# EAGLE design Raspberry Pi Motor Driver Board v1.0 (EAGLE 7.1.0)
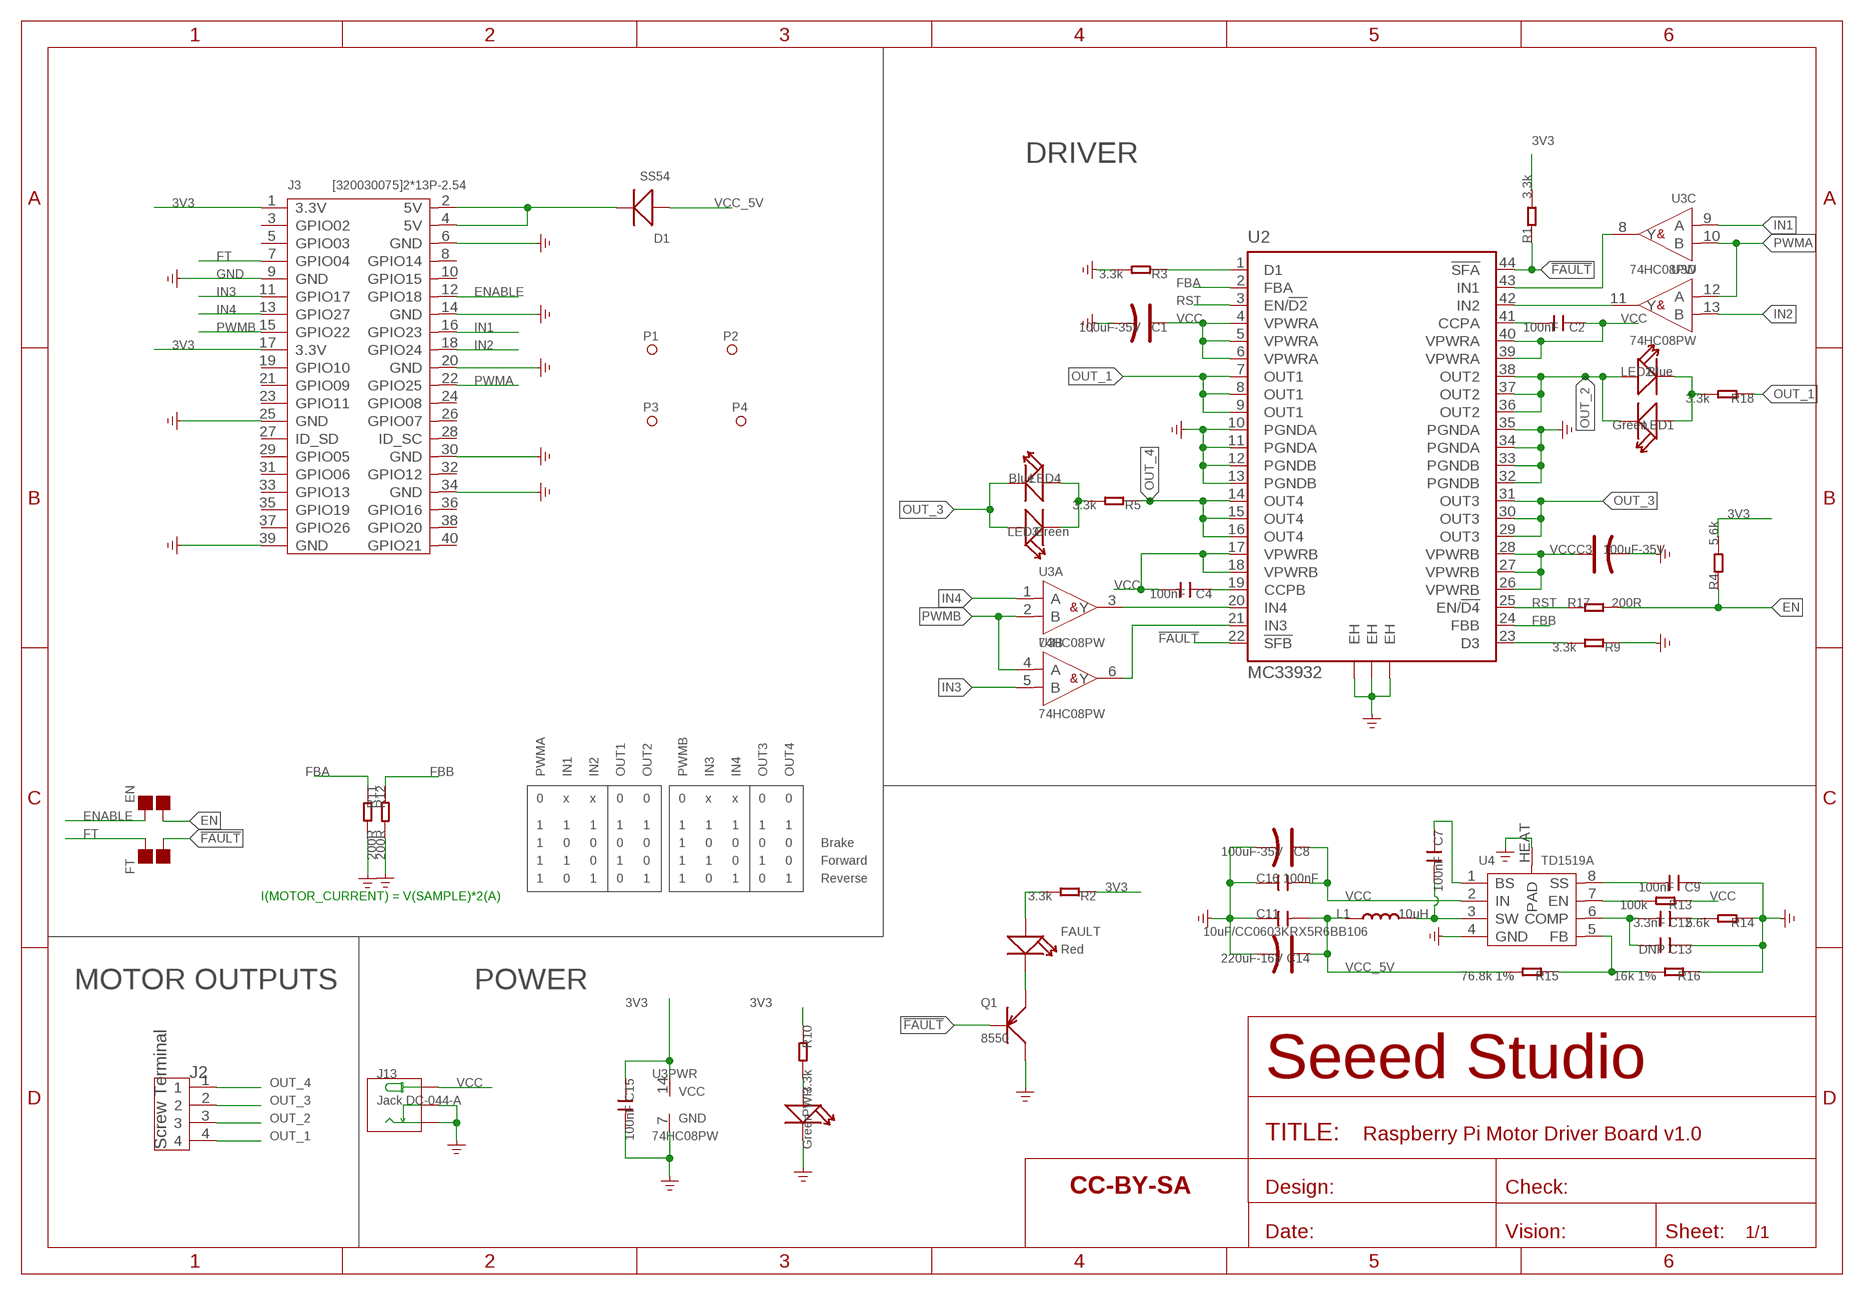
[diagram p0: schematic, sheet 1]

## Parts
C1  100uF-35V  CAP-ELECTRO-E  [ELECTRO-SMD-E-7.8MM]
C2  100nF  C-0603  [C0603]
C3  100uF-35V  CAP-ELECTRO-E  [ELECTRO-SMD-E-7.8MM]
C4  100nF  C-0603  [C0603]
C7  100nF  C-0603  [C0603]
C8  100uF-35V  CAP-ELECTRO-E  [ELECTRO-SMD-E-7.8MM]
C9  100nF  C-0603  [C0603]
C11  10uF/CC0603KRX5R6BB106  C-0603  [C0603]
C12  3.3nF  C-0603  [C0603]
C13  DNP  C-0603  [C0603]
C14  220uF-16V  CAP-ELECTRO-D  [ELECTRO-SMD-D-5.6MM]
C15  100nF  C-0603  [C0603]
C16  100nF  C-0603  [C0603]
D1  SS54  DIODESMB  [DO_214AA]
EN  PAD-JUMPER-2P  [2P-SMD-1.78X1.27]
FAULT  Red  LED'0603'  [LED-0603]
FT  PAD-JUMPER-2P  [2P-SMD-1.78X1.27]
J2  Screw Terminal  SCREW-TERMINAL-4P'3.5'  [4P-3.5]
J3  [320030075]2*13P-2.54  HEADER-2X20P  [2X20P-2.54-65/35MIL]
J13  Jack DC-044-A  JACK-DC-044  [DC-044]
L1  10uH  L'0630'  [L0630]
LED1  Green  LED'0603'  [LED-0603]
LED2  Blue  LED'0603'  [LED-0603]
LED3  Green  LED'0603'  [LED-0603]
LED4  Blue  LED'0603'  [LED-0603]
P1  PAD-MARK'ANNULAR'  [ROUND-MARK-1.0]
P2  PAD-MARK'ANNULAR'  [ROUND-MARK-1.0]
P3  PAD-MARK'ANNULAR'  [ROUND-MARK-1.0]
P4  PAD-MARK'ANNULAR'  [ROUND-MARK-1.0]
PWR  Green  LED'0603'  [LED-0603]
Q1  8550  TRANSISTOR-PNP-SOT23  [SOT-23]
R1  3.3k  R-0603  [R0603]
R2  3.3k  R-0603  [R0603]
R3  3.3k  R-0603  [R0603]
R4  5.6k  R-0603  [R0603]
R5  3.3k  R-0603  [R0603]
R9  3.3k  R-0603  [R0603]
R10  3.3k  R-0603  [R0603]
R11  200R  R-0603  [R0603]
R12  200R  R-0603  [R0603]
R13  100k  R-0603  [R0603]
R14  5.6k  R-0603  [R0603]
R15  76.8k 1%  R-0603  [R0603]
R16  16k 1%  R-0603  [R0603]
R17  200R  R-0603  [R0603]
R18  3.3k  R-0603  [R0603]
U2  MC33932  [HSOP44]
U3  74HC08PW  [TSSOP14]
U4  TD1519A  TD1484A  [SOP8-W/HEAT]
U$12  SEEEDSTUDIO-OPEN-SCH-FRAME  [SEEEDSTUDIO-PCB-FRAME]

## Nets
3V3: C15.1 J3.1(3.3V) J3.17(3.3V) R1.2 R2.1 R4.2 R10.1 U3.14(PWR:VCC)
!FAULT: FT.1 Q1.1(B) R1.1 U2.22(!SFB) U2.44(!SFA)
EN: EN.1 R4.1 R17.2
ENABLE: EN.2 J3.12(GPIO18)
FBA: R11.1 U2.2(FBA)
FBB: R12.1 U2.24(FBB)
FT: FT.2 J3.7(GPIO04)
GND: C1.- C3.- C8.- C9.1 C11.1 C13.1 C14.- C15.2 C16.1 J3.6(GND) J3.9(GND) J3.14(GND) J3.20(GND) J3.25(GND) J3.30(GND) J3.34(GND) J3.39(GND) J13.- J13.CDN PWR.- Q1.3(C) R3.2 R9.1 R11.2 R12.2 R14.1 R16.1 U2.10(PGNDA) U2.11(PGNDA) U2.12(PGNDB) U2.13(PGNDB) U2.32(PGNDB) U2.33(PGNDB) U2.34(PGNDA) U2.35(PGNDA) U2.EH@1(EH) U2.EH@2(EH) U2.EH@3(EH) U3.7(PWR:GND) U4.4(GND) U4.HEAT(PAD) ; supply symbol labelled GND_POWER
IN1: J3.16(GPIO23) U3.9(C:A)
IN2: J3.18(GPIO24) U3.13(D:B)
IN3: J3.11(GPIO17) U3.5(B:B)
IN4: J3.13(GPIO27) U3.1(A:A)
N$1: FAULT.- Q1.2(E)
N$2: FAULT.+ R2.2
N$3: D1.2(-) J3.2(5V) J3.4(5V)
N$4: R3.1 U2.1(D1)
N$6: U2.21(IN3) U3.6(B:Y)
N$8: LED3.- LED4.+ R5.2
N$11: C7.2 L1.2 U4.3(SW)
N$12: U2.42(IN2) U3.11(D:Y)
N$14: LED1.+ LED2.- R18.2
N$15: R15.1 R16.2 U4.5(FB)
N$16: R9.2 U2.23(D3)
N$17: C9.2 U4.8(SS)
N$18: R13.2 U4.7(EN)
N$19: C7.1 U4.1(BS)
N$20: C12.2 C13.2 U4.6(COMP)
N$23: U2.43(IN1) U3.8(C:Y)
N$25: C12.1 R14.2
N$26: U2.20(IN4) U3.3(A:Y)
N$28: C2.2 U2.41(CCPA)
N$30: C4.1 U2.19(CCPB)
N$54: PWR.+ R10.2
OUT_1: J2.4 R18.1 U2.7(OUT1) U2.8(OUT1) U2.9(OUT1)
OUT_2: J2.3 LED1.- LED2.+ U2.36(OUT2) U2.37(OUT2) U2.38(OUT2)
OUT_3: J2.2 LED3.+ LED4.- U2.29(OUT3) U2.30(OUT3) U2.31(OUT3)
OUT_4: J2.1 R5.1 U2.14(OUT4) U2.15(OUT4) U2.16(OUT4)
PWMA: J3.22(GPIO25) U3.10(C:B) U3.12(D:A)
PWMB: J3.15(GPIO22) U3.2(A:B) U3.4(B:A)
RST: R17.1 U2.3(EN/!D2) U2.25(EN/!D4)
VCC: C1.+ C2.1 C3.+ C4.2 C8.+ C16.2 J13.+ R13.1 U2.4(VPWRA) U2.5(VPWRA) U2.6(VPWRA) U2.17(VPWRB) U2.18(VPWRB) U2.26(VPWRB) U2.27(VPWRB) U2.28(VPWRB) U2.39(VPWRA) U2.40(VPWRA) U4.2(IN)
VCC_5V: C11.2 C14.+ D1.1(+) L1.1 R15.2
Unconnected: J3.3(GPIO02) J3.5(GPIO03) J3.8(GPIO14) J3.10(GPIO15) J3.19(GPIO10) J3.21(GPIO09) J3.23(GPIO11) J3.24(GPIO08) J3.26(GPIO07) J3.27(ID_SD) J3.28(ID_SC) J3.29(GPIO05) J3.31(GPIO06) J3.32(GPIO12) J3.33(GPIO13) J3.35(GPIO19) J3.36(GPIO16) J3.37(GPIO26) J3.38(GPIO20) J3.40(GPIO21)

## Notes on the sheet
- DRIVER
- PWMA | IN1 | IN2 | OUT1 | OUT2 | PWMB | IN3 | IN4 | OUT3 | OUT4
- 0 | x | x | 0 | 0 | 0 | x | x | 0 | 0
- 1 | 1 | 1 | 1 | 1 | 1 | 1 | 1 | 1 | 1
- 1 | 0 | 0 | 0 | 0 | 1 | 0 | 0 | 0 | 0 | Brake
- 1 | 1 | 0 | 1 | 0 | 1 | 1 | 0 | 1 | 0 | Forward
- 1 | 0 | 1 | 0 | 1 | 1 | 0 | 1 | 0 | 1 | Reverse
- I(MOTOR_CURRENT) = V(SAMPLE)*2(A)
- MOTOR OUTPUTS | POWER

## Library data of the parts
C1 C3 C8 C14 = Discrete:CAP*: Electrolytic Capacitors,Tantalum Capacitors and Super Capacitors
C2 C4 C7 C9 C11-C13 C15 C16 = Discrete:C*: Ceramic Capacitors
D1 = Discrete-new:DIODE*
EN FT = Discrete:PAD-JUMPER-2P; PARTNO: DNP
FAULT LED1-LED4 PWR = Discrete:LED*
J2 = Connector :SCREW-TERMINAL-4P
J3 = Connector-new:HEADER-2X20P
J13 = Connector :JACK-DC-044
L1 = Discrete:L*
P1-P4 = Discrete-new:PAD-MARK; PARTNO: DNP
Q1 = Discrete-new:TRANSISTOR-PNP*: PNP audion
R1-R5 R9-R18 = Discrete:R*
U2 = template:MC33932: 5.0 A Throttle Control H-Bridge Auto generated by make-symbol-device-package-bsdl.ulp Rev. 33 Source: http://www.freescale.com/files/analog/doc/data_sheet/MC33932.pdf?fpsp=1; MPN: MC33932VW; OC_FARNELL: 1701639; OC_NEWARK: 67P3304
U3 = template :74*08: Quad 2-input AND gate
U4 = template:TD1484A: The TD1484 is a monolithic synchronous buck regulator. The device integrates two 90mΩ MOSFETs, and provides 3A of continuous load current over a wide input voltage of 4.75V to 23V. Current mode control provides fast transient response and cycle-by-cycle current limit. An adjustable soft-start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
U$12 = moudle-new:SEEEDSTUDIO-OPEN-SCH-FRAME

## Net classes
0 default: width 0.076 mm, drill 0.102 mm, clearance 0.076 mm
1 vcc: width 5.08 mm, clearance 0.254 mm

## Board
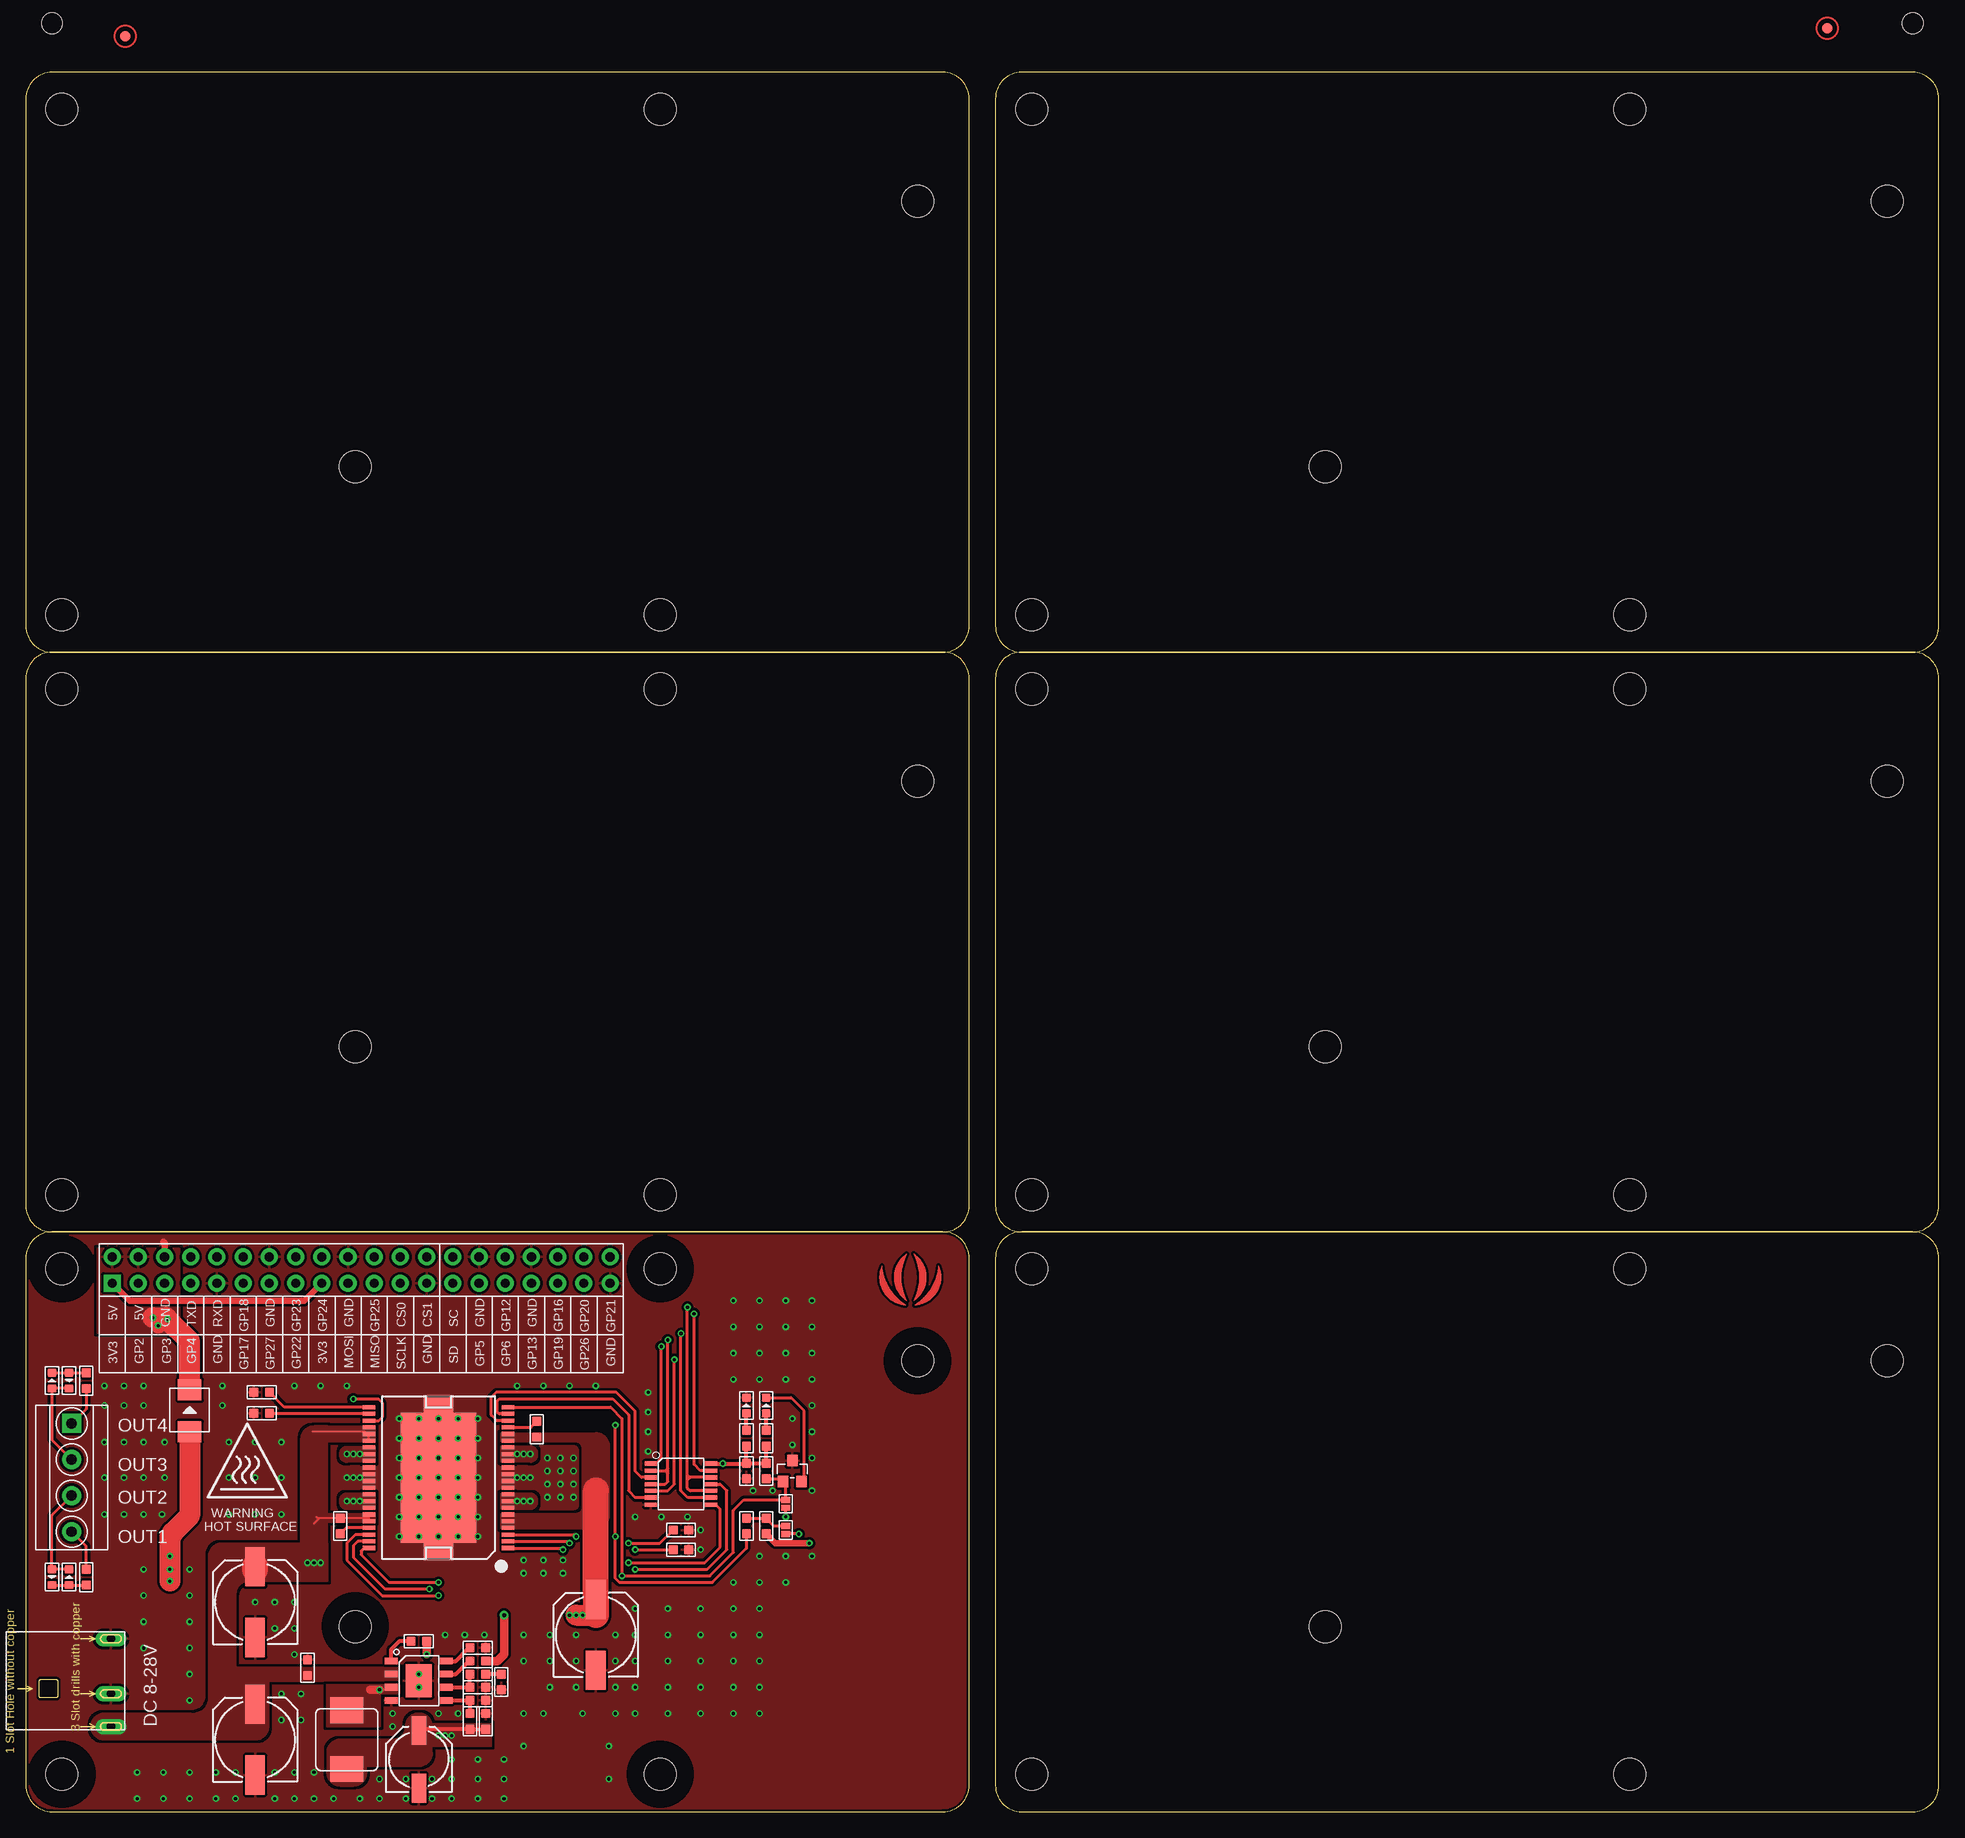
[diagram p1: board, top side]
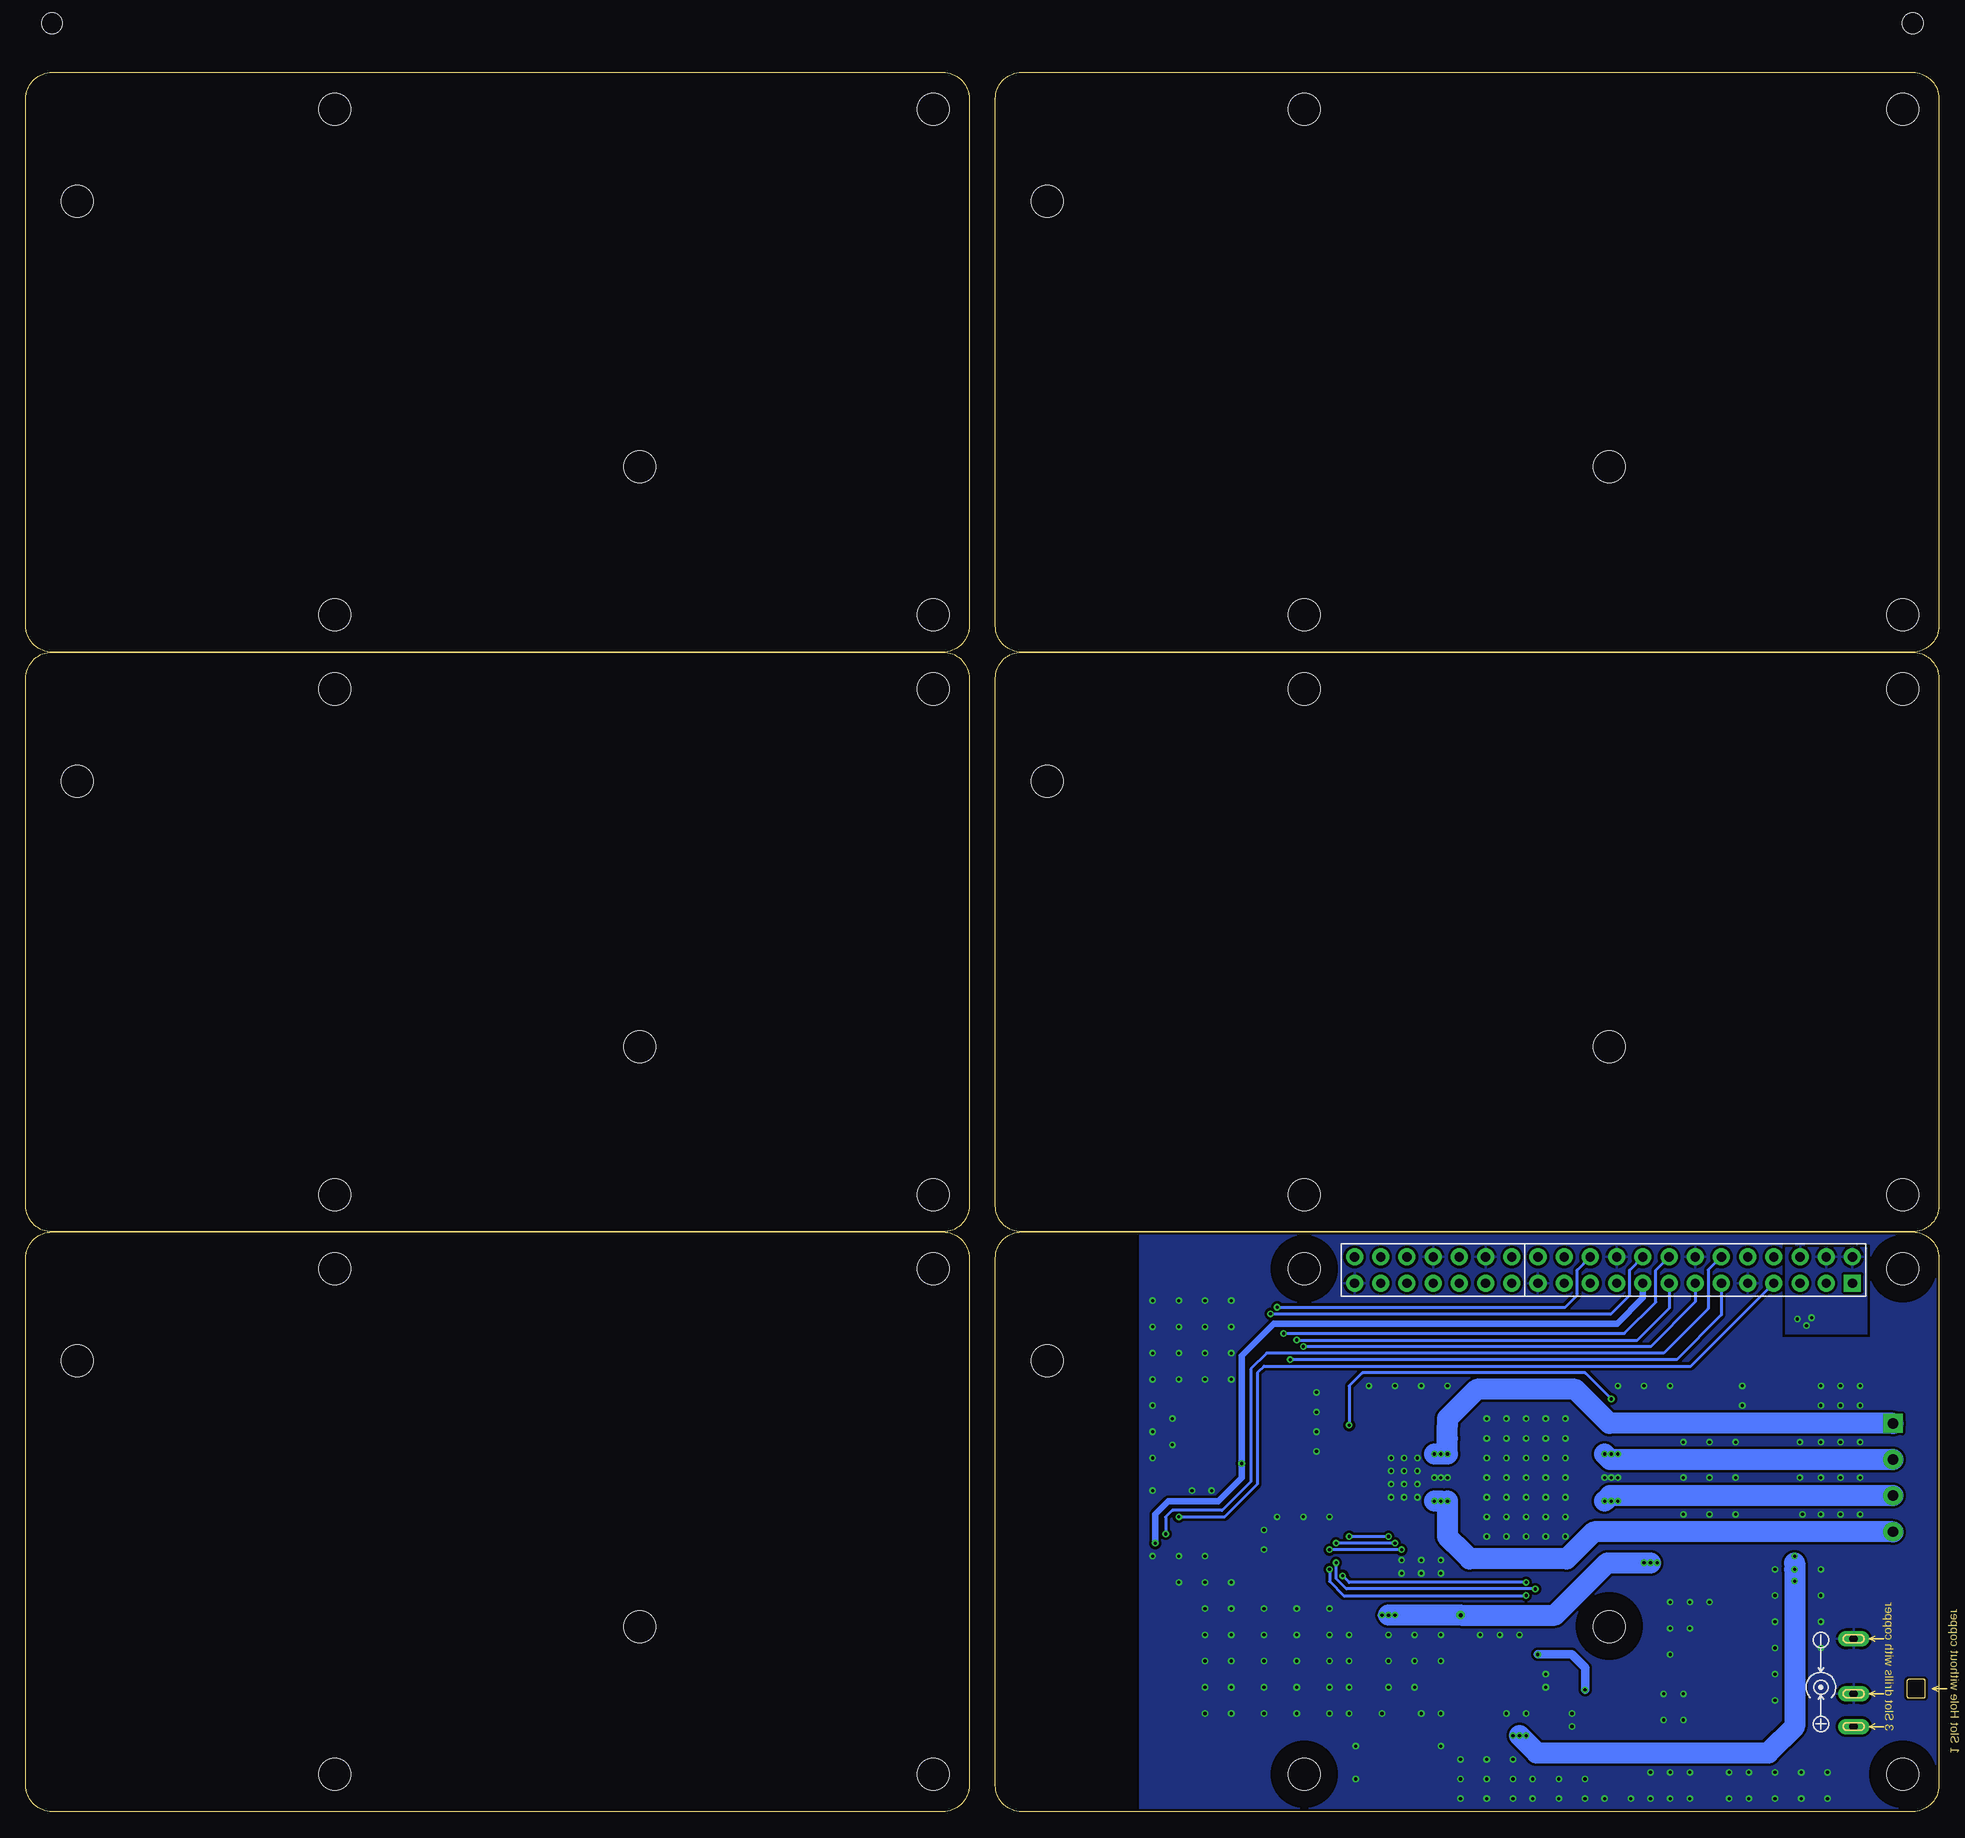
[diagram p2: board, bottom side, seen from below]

Size 185.42 x 168.59 mm. Coordinates in mm from the lower left corner, seen from the top.
Copper layers (1*16): Top 0.035mm / dielectric 1.5mm / Bottom 0.035mm
Design rules "SeeedStudio_2layer_DRU_no_angle_20140221 *": minimum track width 6mil, minimum drill 12mil, track to track 6mil, track to pad 6mil, pad to pad 6mil, via to via 6mil, smd to smd 0mil, copper to edge 10mil, drill to drill 10mil, minimum pad ring 10mil, minimum via ring 6mil, stop-mask expansion 2mil, vias tented up to drill 25mil, thermal gap 10mil
Holes 2.03 mm at 2.54,-4.45 182.88,-4.45 182.88,173.35 2.54,173.35

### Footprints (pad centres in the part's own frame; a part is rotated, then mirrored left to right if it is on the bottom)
ELECTRO-SMD-E-7.8MM = smd 3.81 x 1.905: + 3.429,0; - -3.429,0
C0603 = smd 0.889 x 0.889: 1 -0.762,0; 2 0.762,0
ELECTRO-SMD-D-5.6MM = smd 2.794 x 1.397: + 2.794,0; - -2.794,0
DO_214AA = smd 2.032 x 2.286: 1 -2.032,0; 2 2.032,0
2P-SMD-1.78X1.27 = smd 0.889 x 0.61: 1 0,0.381; 2 0,-0.381
LED-0603 = smd 0.762 x 0.889: + -0.762,0; - 0.762,0
4P-3.5 = drill 1 pad 1.85 square: 1 -5.25,0 | drill 1 pad 1.85: 2 -1.75,0; 3 1.75,0; 4 5.25,0
2X20P-2.54-65/35MIL = drill 0.889 pad 1.651 square: 1 1.27,24.13 | drill 0.889 pad 1.651: 2 -1.27,24.13; 3 1.27,21.59; 4 -1.27,21.59; 5 1.27,19.05; 6 -1.27,19.05; 7 1.27,16.51; 8 -1.27,16.51; 9 1.27,13.97; 10 -1.27,13.97; 11 1.27,11.43; 12 -1.27,11.43; 13 1.27,8.89; 14 -1.27,8.89; 15 1.27,6.35; 16 -1.27,6.35; 17 1.27,3.81; 18 -1.27,3.81; 19 1.27,1.27; 20 -1.27,1.27; 21 1.27,-1.27; 22 -1.27,-1.27; 23 1.27,-3.81; 24 -1.27,-3.81; 25 1.27,-6.35; 26 -1.27,-6.35; 27 1.27,-8.89; 28 -1.27,-8.89; 29 1.27,-11.43; 30 -1.27,-11.43; 31 1.27,-13.97; 32 -1.27,-13.97; 33 1.27,-16.51; 34 -1.27,-16.51; 35 1.27,-19.05; 36 -1.27,-19.05; 37 1.27,-21.59; 38 -1.27,-21.59; 39 1.27,-24.13; 40 -1.27,-24.13
DC-044 = drill 0.813 pad 1.524 long: + 3.175,10.16; - -5.334,10.16; CDN 0,10.16
L0630 = smd 2.5 x 3.2: 1 -2.85,0; 2 2.85,0
ROUND-MARK-1.0 = smd 1.016 x 1.016: P$1 0,0
SOT-23 = smd 1.016 x 1.143: 1 -0.889,-1.016; 2 0.889,-1.016; 3 0,1.016
R0603 = smd 0.889 x 0.889: 1 -0.762,0; 2 0.762,0
HSOP44 = smd 0.4 x 1.2: 1 -6.825,-6.75; 2 -6.175,-6.75; 3 -5.525,-6.75; 4 -4.875,-6.75; 5 -4.225,-6.75; 6 -3.575,-6.75; 7 -2.925,-6.75; 8 -2.275,-6.75; 9 -1.625,-6.75; 10 -0.975,-6.75; 11 -0.325,-6.75; 12 0.325,-6.75; 13 0.975,-6.75; 14 1.625,-6.75; 15 2.275,-6.75; 16 2.925,-6.75; 17 3.575,-6.75; 18 4.225,-6.75; 19 4.875,-6.75; 20 5.525,-6.75; 21 6.175,-6.75; 22 6.825,-6.75; 23 6.825,6.75; 24 6.175,6.75; 25 5.525,6.75; 26 4.875,6.75; 27 4.225,6.75; 28 3.575,6.75; 29 2.925,6.75; 30 2.275,6.75; 31 1.625,6.75; 32 0.975,6.75; 33 0.325,6.75; 34 -0.325,6.75; 35 -0.975,6.75; 36 -1.625,6.75; 37 -2.275,6.75; 38 -2.925,6.75; 39 -3.575,6.75; 40 -4.225,6.75; 41 -4.875,6.75; 42 -5.525,6.75; 43 -6.175,6.75; 44 -6.825,6.75 | smd 12.6 x 7.3: EH@1 0,0 | smd 1.7 x 2.9: EH@2 -7.15,0; EH@3 7.15,0
TSSOP14 = smd 0.4 x 1.2: 1 -2,-2.925; 2 -1.3,-2.925; 3 -0.65,-2.925; 4 0,-2.925; 5 0.65,-2.925; 6 1.3,-2.925; 7 2,-2.925; 8 2,2.925; 9 1.3,2.925; 10 0.65,2.925; 11 0,2.925; 12 -0.65,2.925; 13 -1.3,2.925; 14 -2,2.925
SOP8-W/HEAT = smd 0.635 x 1.27: 1 -1.905,-2.667; 2 -0.635,-2.667; 3 0.635,-2.667; 4 1.905,-2.667; 5 1.905,2.667; 6 0.635,2.667; 7 -0.635,2.667; 8 -1.905,2.667 | smd 3.175 x 2.54: HEAT 0,0
RASPBERRY-PI-B+/B = hole 3.1: 3.503,52.622; 3.503,3.622; 61.503,52.622; 61.503,3.622; 31.951,17.951; 86.431,43.7

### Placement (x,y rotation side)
C1  55.24,17.14 90 top
C2  30.48,27.69 270 top
C3  22.23,20.32 90 top
C4  49.53,37.08 270 top
C7  38.1,16.51 0 top
C8  22.23,6.99 90 top
C9  43.81,15.88 180 top
C11  44.58,8.76 270 top
C12  43.81,13.34 180 top
C13  43.81,12.06 180 top
C14  38.1,5.08 90 top
C15  69.85,33.02 270 top
C16  27.3,13.97 270 top
D1  15.88,38.86 90 top
EN  73.66,27.3 0 top
FAULT  71.75,39.37 90 top
FT  73.66,29.84 0 top
J2  4.45,32.38 270 top
J3  32.5,52.5 270 bottom
J13  -1.91,11.43 270 top
L1  31.11,6.99 90 top
LED1  4.19,22.73 90 top
LED2  2.54,22.73 270 top
LED3  2.54,41.78 90 top
LED4  4.19,41.78 270 top
P1  not placed on the board
P2  not placed on the board
P3  not placed on the board
P4  not placed on the board
PWR  69.85,39.37 90 top
Q1  74.3,33.02 0 top
R1  71.75,33.02 90 top
R2  71.75,36.2 90 top
R3  63.5,25.4 0 top
R4  71.75,27.69 270 top
R5  5.84,41.78 90 top
R9  22.86,40.64 0 top
R10  69.85,36.2 90 top
R11  63.5,27.3 0 top
R12  22.86,38.61 180 top
R13  43.81,14.61 180 top
R14  46.1,12.57 90 top
R15  43.05,8.76 270 top
R16  43.81,10.79 180 top
R17  69.85,27.69 90 top
R18  5.84,22.73 270 top
U2  40.01,32.38 90 top
U3  63.5,31.75 270 top
U4  38.1,12.7 270 top
U$12  not placed on the board
U$14  [SEEED-COPPER-280*268MIL]  85.72,50.8 0 top
U$27  [RASPBERRY-PI-B+/B]  0,0 0 top
U$29  [RASPBERRY-PI-B+/B]  0,56.2 0 top
U$32  [RASPBERRY-PI-B+/B]  93.98,0 0 top
U$33  [RASPBERRY-PI-B+/B]  0,112.39 0 top
U$34  [RASPBERRY-PI-B+/B]  93.98,56.2 0 top
U$35  [RASPBERRY-PI-B+/B]  93.98,112.39 0 top

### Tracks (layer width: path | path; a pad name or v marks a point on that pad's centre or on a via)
3V3  (via drill 0.3 pad 0.64)
  Top 0.305: U3.14 65.94,33.75
  Top 0.406: U3.14 v67.56,33.75 69.82,33.75 C15.1 | C15.1 R1.2 R2.1 | C15.1 R10.1
  Top 0.61: J3.1 8.4,51.23 10.1,49.53 26.99,49.53 J3.17 | R4.2 72.64,26.04 v75.95,26.04
  Bottom 0.61: J3.17 28.69,49.8 31.18,47.31 64.45,47.31 67.56,44.2 v67.56,33.75 67.56,32.38 69.85,30.1 74.68,30.1 75.95,28.83 v75.95,26.04
!FAULT  (via drill 0.3 pad 0.64)
  Top 0.305: R1.1 73.15,32.26 Q1.1 73.66,31.75 FT.1 69.6,30.23 68.58,29.2 68.58,25.15 66.29,22.86 v57.78,22.86 57.78,38.1 56.67,39.21 U2.22 | v40.01,22.23 35.2,22.23 32.51,24.92 32.51,25.27 32.8,25.56 U2.44
  Bottom 0.305: v40.01,22.23 57.15,22.23 v57.78,22.86
EN
  Top 0.305: R17.2 R4.1 72.52,27.69 EN.1
ENABLE  (via drill 0.3 pad 0.64)
  Top 0.305: v74.93,26.92 EN.2
  Bottom 0.305: J3.12 21.1,53.77 22.35,52.51 22.35,48.77 26.67,44.45 65.15,44.45 66.67,42.93 66.67,32 69.47,29.21 74.3,29.21 74.93,28.57 v74.93,26.92
FBA  (via drill 0.3 pad 0.64)
  Top 0.305: U2.2 52.53,26.21 v52.7,26.04 | v58.42,26.04 61.47,26.04 R11.1
  Bottom 0.305: v52.7,26.04 v58.42,26.04
FBB
  Top 0.305: U2.24 23.67,38.56 R12.1
FT  (via drill 0.3 pad 0.64)
  Top 0.305: v73.66,28.57 FT.2
  Bottom 0.305: v73.66,28.57 69.22,28.57 66.04,31.75 66.04,42.53 65.39,43.18 24.04,43.18 J3.7
GND  (via drill 0.3 pad 0.64)
  Top 0.61: J3.6 13.45,55.13 13.34,55.24
  other vias: 36.2,38.1 40.01,38.1 43.81,38.1 38.1,34.29 36.2,34.29 43.81,34.29 36.2,26.67 38.1,26.67 38.1,32.38 43.81,32.38 40.01,34.29 36.2,32.38 31.75,32.38 32.38,32.38 48.9,32.38 47.62,32.38 38.1,38.1 41.91,38.1 36.2,36.2 38.1,36.2 40.01,36.2 41.91,36.2 43.81,36.2 36.2,30.48 36.2,28.57 40.01,26.67 41.91,26.67 43.81,26.67 38.1,30.48 41.91,34.29 41.91,32.38 40.01,32.38 40.01,30.48 41.91,30.48 43.81,30.48 38.1,28.57 40.01,28.57 41.91,28.57 43.81,28.57 74.3,35.56 74.3,38.1 11.43,39.37 11.43,41.27 9.53,41.27 9.53,39.37 7.62,39.37 7.62,41.27 26.04,41.27 28.57,41.27 31.11,41.27 60.33,34.92 60.33,36.83 60.33,38.73 60.33,40.64 59.05,17.14 62.23,17.14 65.41,17.14 57.15,9.53 59.05,9.53 53.98,9.53 59.05,19.68 62.23,19.68 65.41,19.68 57.15,14.61 59.05,14.61 59.05,12.06 57.15,12.06 68.58,49.53 68.58,46.99 68.58,44.45 68.58,41.91 71.12,41.91 71.12,44.45 71.12,46.99 71.12,49.53 73.66,49.53 73.66,46.99 73.66,44.45 73.66,41.91 68.58,22.23 68.58,19.68 65.41,9.53 68.58,17.14 71.12,24.77 71.12,22.23 71.12,19.68 62.23,9.53 71.12,17.14 68.58,14.61 71.12,14.61 71.12,12.06 68.58,12.06 31.11,32.38 48.26,32.38 65.41,25.4 65.41,27.3 73.66,22.23 19.05,39.37 19.05,41.27 47.62,41.27 50.16,41.27 52.7,41.27 55.24,41.27 59.05,28.57 61.59,28.57 64.14,28.57 38.1,13.34 38.1,12.06 35.56,9.53 35.56,8.26 41.91,9.53 40.01,9.53 26.04,15.24 26.04,17.78 26.04,20.32 24.13,20.32 24.13,17.78 24.77,11.43 26.67,11.43 26.67,8.89 24.77,8.89 13.21,28.83 19.68,28.83 22.23,28.83 24.77,28.83 13.46,32.38 19.68,32.38 22.23,32.38 24.77,32.38 24.77,35.81 22.23,35.81 19.68,35.81 13.46,35.81 15.88,23.5 15.88,20.95 15.88,18.41 15.88,15.88 15.88,13.34 15.88,10.79 11.43,35.81 9.53,35.81 7.62,35.81 7.62,32.38 9.53,32.38 11.43,32.38 11.43,28.83 9.53,28.83 7.62,28.83 11.43,23.5 11.43,20.95 11.43,18.41 18.41,3.81 15.88,3.81 13.34,3.81 20.32,3.81 24.13,3.81 10.79,3.81 10.79,1.27 13.34,1.27 15.88,1.27 18.41,1.27 20.32,1.27 24.13,1.27 26.04,3.81 26.04,1.27 27.94,1.27 27.94,3.81 11.43,15.88 36.83,1.27 36.83,3.17 34.29,3.17 34.29,1.27 32.38,1.27 29.84,1.27 39.37,3.17 39.37,1.27 41.27,3.17 41.27,1.27 41.27,5.08 43.81,5.08 46.35,5.08 46.35,3.17 43.81,3.17 43.81,1.27 46.35,1.27 53.34,17.14 48.26,17.14 48.26,14.61 50.8,14.61 44.45,17.14 42.55,17.14 40.64,17.14 53.34,12.06 53.34,14.61 50.8,12.06 50.16,9.53 48.26,9.53 48.26,6.35 62.23,12.06 62.23,14.61 65.41,14.61 65.41,12.06 50.55,34.29 51.82,34.29 53.09,34.29 53.09,33.02 51.82,33.02 50.55,33.02 50.55,31.75 51.82,31.75 53.09,31.75 53.09,30.48 51.82,30.48 50.55,30.48 50.8,17.14 57.15,17.14 68.58,9.53 71.12,9.53 48.26,24.38 50.16,24.38 52.07,24.38 48.26,23.11 50.16,23.11 52.07,23.11 73.66,24.77 76.2,24.77 76.2,49.53 76.2,46.99 76.2,44.45 76.2,41.91 76.2,39.37 76.2,36.83 76.2,34.29 56.52,6.35 56.52,3.17 22.23,20.32 70.48,31.11 72.39,31.11 76.2,31.11
  pour Top (isolate 0.254, rank 3, no thermals): 37.47,33.4 31.11,33.4 arc90 30.48,32.77 30.48,32 arc90 31.11,31.37 37.47,31.31
  pour Top (isolate 0.254, rank 3, no thermals): 42.48,33.4 42.48,31.37 48.83,31.37 arc90 49.47,32 49.47,32.77 arc90 48.83,33.4
  pour Top (isolate 0.254, rank 3): 0,55.88 92.2,55.88 92.08,0 0,0
  pour Bottom (isolate 0.254, rank 3): 0,55.88 77.47,55.88 77.47,0 0,0
  pour Top (isolate 0.254, no thermals): 35.56,40.64 44.45,40.64 44.45,24.13 35.56,24.13
IN1  (via drill 0.3 pad 0.64)
  Top 0.305: U3.9 64.17,30.45 63.5,31.11 v63.5,46.35
  Bottom 0.305: J3.16 27.43,52.49 27.43,49.4 30.48,46.35 v63.5,46.35
IN2  (via drill 0.3 pad 0.64)
  Top 0.305: U3.13 65.38,33.05 64.77,33.66 v64.77,48.26
  Bottom 0.305: v64.77,48.26 31.77,48.26 29.97,50.06 29.97,52.49 J3.18
IN3  (via drill 0.3 pad 0.64)
  Top 0.305: U3.5 62.22,31.1 62.87,31.75 v62.87,43.81
  Bottom 0.305: v62.87,43.81 25.4,43.81 21.07,48.15 J3.11
IN4  (via drill 0.3 pad 0.64)
  Top 0.305: U3.1 61.05,33.75 61.59,34.29 v61.59,45.09
  Bottom 0.305: v61.59,45.09 27.94,45.09 23.61,49.41 J3.13
N$1
  Top 0.305: Q1.2 75.44,32 75.44,38.86 74.17,40.13 FAULT.-
N$2
  Top 0.406: R2.2 FAULT.+
N$3  (via drill 0.3 pad 0.64)
  Top 1.524: 13.97,47.37 13.46,47.88 13.59,47.88 | v13.72,47.75 13.46,47.75 v12.83,47.12
  Top 2.032: v12.32,47.88 13.59,47.88 v13.72,47.75 15.88,45.59 D1.2
  pour Bottom (isolate 0.254): 6.99,54.61 14.86,54.61 14.86,46.35 6.99,46.35
  pour Top (isolate 0.254): 6.99,54.61 14.86,54.61 14.86,46.35 6.99,46.35
N$4  (via drill 0.3 pad 0.64)
  Top 0.305: U2.1 51.91,25.56 v52.07,25.4 | v59.05,25.4 R3.1
  Bottom 0.305: v52.07,25.4 v59.05,25.4
N$6
  Top 0.305: U2.21 45.9,38.56 45.72,38.73 45.72,39.83 45.9,40.01 56.89,40.01 58.42,38.48 58.42,31.11 59.09,30.45 U3.6
N$8
  Top 0.305: LED3.- LED4.+ R5.2
N$11  (via drill 0.3 pad 0.64)
  Top 0.813: C7.2 v38.86,15.24 | v34.29,11.81 33.4,11.81
  Bottom 0.813: v38.86,15.24 35.56,15.24 34.29,13.97 v34.29,11.81
  pour Top (isolate 0.254, no thermals): 29.21,12.32 36.2,12.32 36.2,11.43 34.29,11.43 34.29,8.26 29.21,8.26
N$12  (via drill 0.3 pad 0.64)
  Top 0.305: v59.05,23.5 66.04,23.5 67.94,25.4 67.94,31.11 67.31,31.75 U3.11 | U2.42 31.94,26.86 31.11,26.04 31.11,24.39 34.55,20.95 v40.01,20.95
  Bottom 0.305: v59.05,23.5 59.05,22.33 57.68,20.95 v40.01,20.95
N$14
  Top 0.305: LED2.- LED1.+ R18.2
N$15
  Top 0.406: U4.5 R16.2 R15.1
N$16
  Top 0.305: U2.23 25.05,39.21 R9.2
N$17
  Top 0.406: U4.8 41.66,14.61 42.93,15.88 C9.2
N$18
  Top 0.406: U4.7 41.66,13.34 42.93,14.61 R13.2
N$19
  Top 0.406: C7.1 36.2,16.51 35.43,15.75 U4.1
N$20
  Top 0.406: U4.6 C13.2 C12.2
N$23  (via drill 0.3 pad 0.64)
  Top 0.305: v58.42,24.13 65.79,24.13 67.31,25.65 67.31,29.34 66.9,29.75 U3.8 | U2.43 32.18,26.21 31.75,25.78 31.75,24.65 34.81,21.59 v39.12,21.59
  Bottom 0.305: v39.12,21.59 57.43,21.59 58.42,22.58 v58.42,24.13
N$25
  Top 0.406: R14.2 C12.1
N$26
  Top 0.305: U3.3 59.67,32.4 59.05,33.02 59.05,38.84 57.25,40.64 45.59,40.64 45.09,40.13 45.09,38.48 45.15,38.42 45.66,37.91 U2.20
N$28
  Top 0.305: U2.41 31.07,27.51 C2.2
N$30
  Top 0.305: U2.19 48.94,37.26 C4.1
N$54
  Top 0.406: R10.2 PWR.+
OUT_1  (via drill 0.3 pad 0.64)
  Top 0.305: R18.1 5.84,25.74 J2.4
  Bottom 2.032: v48.9,30.1 v48.26,30.1 v47.62,30.1 47.62,26.67 46.04,25.08 45.47,24.51 36.07,24.51 33.44,27.14 J2.4
  pour Top (isolate 0.254, rank 2, no thermals): 46.1,30.86 48.9,30.86 arc-90 49.53,30.23 49.53,29.97 arc-90 48.9,29.34 46.1,29.34
OUT_2  (via drill 0.3 pad 0.64)
  Top 0.305: LED1.- LED2.+ 2.54,28.73 J2.3
  Bottom 2.032: J2.3 31.85,30.64 v32.38,30.1
  other vias: 31.75,30.1 31.11,30.1
  pour Top (isolate 0.254, rank 2, no thermals): 33.85,30.86 33.85,29.34 31.11,29.34 arc-90 30.48,29.97 30.48,30.23 arc-90 31.11,30.86
OUT_3  (via drill 0.3 pad 0.64)
  Top 0.305: J2.2 2.54,36.04 LED3.+ LED4.-
  Bottom 2.032: J2.2 31.85,34.13 v32.38,34.67
  other vias: 31.75,34.67 31.11,34.67
  pour Top (isolate 0.254, rank 2, no thermals): 33.85,35.37 33.85,33.91 31.11,33.91 arc-90 30.48,34.54 30.48,34.73 arc-90 31.11,35.37
OUT_4  (via drill 0.3 pad 0.64)
  Top 0.305: R5.1 5.84,39.03 J2.1
  Bottom 2.032: v48.9,34.67 v47.62,34.67 47.62,36.2 47.62,37.47 47.62,38.1 44.78,40.95 35.23,40.95 31.92,37.63 J2.1
  other vias: 48.26,34.67
  pour Top (isolate 0.254, rank 2, no thermals): 46.1,33.91 46.1,35.43 48.9,35.43 arc-90 49.53,34.8 49.53,34.54 arc-90 48.9,33.91
PWMA  (via drill 0.3 pad 0.64)
  Top 0.305: U3.10 64.4,31.1 64.14,31.37 64.14,32.13 | 64.14,32.38 64.14,32.64 | 64.14,32.64 v64.14,48.9 | U3.12 64.4,32.4 | 64.37,32.4 64.15,32.4 64.14,32.38 | 64.14,32.13 64.14,32.38 | 64.4,32.4 64.37,32.4 | 64.37,32.4 64.14,32.64 | 64.4,32.4 64.14,32.13
  Bottom 0.305: v64.14,48.9 36.22,48.9 35.05,50.07 35.05,52.49 J3.22
PWMB  (via drill 0.3 pad 0.64)
  Top 0.305: U3.4 61.98,31.75 62.23,32 62.23,32.83 | 62.23,32.83 62.23,33.02 | 62.23,33.02 62.23,33.27 | 62.23,33.27 v62.23,45.72 | U3.2 62.01,33.05 | 62.01,33.05 62.2,33.05 62.23,33.02 | 62.01,33.05 62.23,33.27 | 62.01,33.05 | 62.01,33.05 62.23,32.83
  Bottom 0.305: v62.23,45.72 29.21,45.72 26.15,48.78 J3.15
RST  (via drill 0.3 pad 0.64)
  Top 0.305: v31.75,40.01 34.16,40.01 34.54,39.62 34.54,38.23 34.23,37.91 U2.25 | U2.3 53.15,26.86 v53.34,26.67 | v57.15,37.47 v57.15,26.67 57.15,22.61 57.53,22.23 66.55,22.23 69.85,25.53 R17.1
  Bottom 0.305: v53.34,26.67 v57.15,26.67 | v31.75,40.01 34.29,42.55 55.88,42.55 57.15,41.27 v57.15,37.47
VCC  (via drill 0.3 pad 0.64, 0.38 pad 0.81)
  Top 0.203: U2.28 33.26,36.47 32.89,36.83 27.81,36.83 | U2.40 33.26,28.43 33.27,28.45 28.45,28.45 | 28.45,28.45 28.32,28.45 28.19,28.57 | 27.94,27.94 28.45,28.45
  Top 0.813: R13.1 45.72,14.61 46.35,15.24 v46.35,19.05
  Top 2.032: v53.34,19.05 55.24,19.05
  Top 2.54: 22.23,23.5 C3.+ | 55.24,19.05 C1.+ 55.24,31.11
  Bottom 0.813: v53.34,19.05 v53.98,19.05
  Bottom 2.032: v27.94,24.13 32.13,24.13 37.21,19.05 v46.35,19.05 v52.7,19.05 v53.34,19.05
  other vias: 27.3,24.13 28.57,24.13
  pour Top (isolate 0.254, no thermals): 33.85,37.34 33.85,35.88 29.21,35.88 29.21,37.34
  pour Top (isolate 0.254, no thermals): 33.85,28.89 33.85,28.07 29.21,28.07 29.21,28.89
  pour Top (isolate 0.254, no thermals): 46.1,27.43 46.1,28.89 53.4,28.89 arc90 53.98,29.46 53.98,35.24 arc90 53.34,35.88 46.1,35.88 46.1,36.7 55.24,36.7 arc-90 56.52,35.43 56.52,28.7 arc-90 55.24,27.43
  pour Top (isolate 0.254, no thermals): 29.21,37.34 27.94,37.34 arc90 26.67,36.07 26.67,24.77 29.21,24.77
  pour Top (isolate 0.254, rank 2, no thermals): 36.2,12.7 36.2,13.97 18.41,13.97 18.41,12.7
  pour Top (isolate 0.254, no thermals): 6.35,8.26 arc-90 7.62,9.53 15.88,9.53 arc90 17.78,10.79 17.78,24.77 arc-90 19.05,26.04 29.21,26.04 29.21,22.35 21.59,22.35 arc90 20.32,21.08 20.32,13.97 23.5,13.97 23.5,8.26 arc-90 22.23,6.99 7.62,6.99 arc-90
VCC_5V  (via drill 0.3 pad 0.64)
  Top 0.406: 44.7,8.13 C11.2 R15.2 38.23,8 C14.+ 37.97,7.75
  Top 2.032: D1.1 15.88,28.7 14.22,27.05 14.22,26.92 13.97,26.67 v13.97,23.5 v13.97,22.35
  Bottom 0.203: 13.97,24.13 v13.97,24.77
  Bottom 2.032: 13.97,24.13 v13.97,23.5 13.97,8.26 16.51,5.71 38.99,5.71 v40.64,7.37
  other vias: 41.27,7.37 40.01,7.37
  pour Top (isolate 0.254, no thermals): 29.21,5.71 29.21,3.81 arc90 30.48,2.54 31.75,2.54 arc90 33.02,3.81 33.02,4.45 38.1,4.45 arc90 39.37,5.71 39.37,8.26 arc90 38.1,9.53 arc90 36.83,8.26 arc-90 35.56,6.99 30.48,6.99 arc90
  pour Top (isolate 0.254, no thermals): 38.73,8.51 45.09,8.51 45.09,6.35 38.73,6.35

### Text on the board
tPlace: 5V | 5V | GND | TXD | RXD | GP18 | GND | GP23 | GP24 | GND | GP25 | CS0 | CS1 | SC | GND | GP12 | GND | GP16 | GP20 | GP21 | 3V3 | GP2 | GP3 | GP4 | GND | GP17 | GP27 | GP22 | 3V3 | MOSI | MISO | SCLK | GND | SD | GP5 | GP6 | GP13 | GP19 | GP26 | GND | OUT4 | OUT3 | OUT2 | WARNING / HOT SURFACE | OUT1 | DC 8-28V
Reference: J1
tDocu: J1

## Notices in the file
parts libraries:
moudle-new: This work is licensed under the Creative Commons Attribution 4.0 International License.
To view a copy of this license,visit:
http://creativecommons.org/licenses/by-sa/4.0
moudle-new: CC-BY-SA
